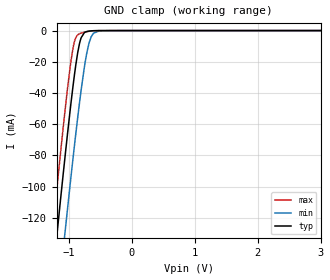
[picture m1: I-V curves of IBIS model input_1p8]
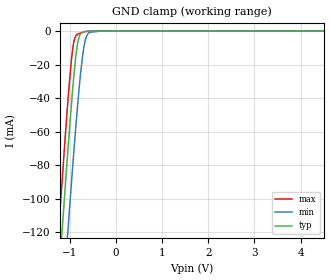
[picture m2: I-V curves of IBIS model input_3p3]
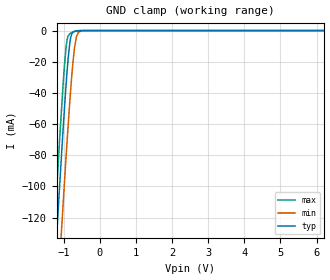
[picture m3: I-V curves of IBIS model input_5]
|Texas Instruments Incorporated
| 12-bit, 8-channel, 1MSPS, SAR ADC with Internal Reference and Internal
| Temperature Sensor
| Marketing part#   Digital Voltage Range   Package-type   #pins
| ADS8028IRTJR   1.65V-5.25V   WQFN   20
| ADS8028IRTJT   1.65V-5.25V   WQFN   20
[IBIS Ver]   4.1
[File name]   ads8028.ibs
[File Rev]   1.0
[Date]   8/3/2015
[Source]
| Texas Instruments Incorporated.
| Analog-eLab Design Center, HPA
| 12500 TI Blvd
| Dallas, TX -75243
[Notes]   Revision History:
| Rev 1.0: 8/3/2015
| - Initial version of the model
| - Model generated from simulations in TISPICE
| - Model matched to SPICE simulation
| - C_comp although listed in numerical order of value are
|   obtained from varying PVT conditions. For PVT conditions for
|   each specific value refer the buffer description under
|   respective [Model]. IBIS model user is responsible for using
|   appropriate C_comp to simulate for Signal Integrity.
[Disclaimer]
| This model is designed as an aid for customers of Texas Instruments.
| TI and its licensors and suppliers make no warranties, either expressed
| or implied, with respect to this  model, including the warranties of
| merchantability or fitness for a particular purpose. The model is
| provided solely on an "as is" basis. The entire risk as to its quality
| and performance is with the customer.
[Copyright]
(C) Copyright 2015 Texas Instruments Incorporated.All rights reserved.
|   ADS8028IRTJ
[Component]   ADS8028IRTJ
[Manufacturer]   TI
[Package]   |20 WQFN - RTJ package
|   typ   min   max
R_pkg   0.06020   0.05752   0.06227
L_pkg   0.91652nH   0.87519nH   0.95139nH
C_pkg   0.12692pF   0.12082pF   0.13078pF
[Pin]  signal_name   model_name   R_pin   L_pin   C_pin
1   AIN3   NC   0.06084   0.93482nH  0.12082pF
2   AIN4   NC   0.05966   0.91410nH  0.12996pF
3   AIN5   NC   0.05964   0.91350nH  0.13005pF
4   AIN6   NC   0.06048   0.92754nH  0.13101pF
5   AIN7   NC   0.06271   0.96574nH  0.12287pF
6   AGND   GND   0.02992   0.59799nH  0.15143pF
7   REF   NC   0.02915   0.57935nH  0.16094pF
8   NC   NC   0.05757   0.87571nH  0.13002pF
9   DGND   GND   0.01969   0.50923nH  0.18030pF
10   AVDD   POWER   0.02967   0.59635nH  0.14994pF
11   _CS   INPUT   0.06227   0.95139nH  0.12238pF
12   TM_BUSY   TRISTATE   0.05995   0.91121nH  0.13014pF
13   DIN   INPUT   0.05966   0.90619nH  0.13006pF
14   DOUT   TRISTATE   0.06040   0.91862nH  0.13078pF
15   SCLK   INPUT   0.06139   0.93650nH  0.12082pF
16   DVDD   POWER   0.06011   0.91724nH  0.11994pF
17   _PD/_RST   INPUT   0.05752   0.87519nH  0.12732pF
18   AIN0   NC   0.05975   0.90986nH  0.12973pF
19   AIN1   NC   0.05767   0.87741nH  0.12809pF
20   AIN2   NC   0.05812   0.88744nH  0.11796pF
|   Model Selectors
[Model Selector] INPUT
input_1p8   1.8V digital Input
input_3p3   3.3V digital Input
input_5   5.0V digital Input
[Model Selector] TRISTATE
tristate_1p8   1.8V digital 3-state
tristate_3p3   3.3V digital 3-state
tristate_5   5.0V digital 3-state
| Models and submodels in the file (6): input_1p8 (Input), input_3p3 (Input), input_5 (Input), tristate_1p8 (3-state), tristate_3p3 (3-state), tristate_5 (3-state)
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|   input_1p8 Model
[Model]   input_1p8
Model_type   Input
Vinl = 0.54
Vinh = 1.26
|   typ   min   max
|   (nom PVT)   (fast PVT)   (slow PVT)
C_comp   4.988e-13   4.299e-13   5.751e-13
[Model spec]
|subparameter
Vinl   0.54   0.495   0.585
Vinh   1.26   1.155   1.365
| Where nom  PVT is Nominal Process, 1.8V, 27C
|   Fast PVT is Strong Process,  1.95V, -40C
|   Slow PVT is Weak Process,   1.65V, 125C
[Voltage Range]   1.8   1.65   1.95
|Junction Temperature
[Temperature Range]   27   125   -40
[Power Clamp Reference]   1.8   1.65   1.95
[GND Clamp Reference]   0   0   0
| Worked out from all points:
|   GND clamp passes 1 mA (typ) near -0.74 V on its own axis
[GND Clamp]
|   Voltage   I(typ)   I(min)   I(max)
-1.8V     -380mA     -425.6mA   -352.6mA
-1.391V   -210.4mA   -258.2mA   -181.1mA
-1.18V    -125.4mA   -174mA     -95.45mA
-1.092V   -91.22mA   -139.8mA   -61.42mA
-1.048V   -74.37mA   -122.7mA   -44.98mA
-937.1mV  -35.3mA    -81.6mA    -11.06mA
-835.2mV  -8.422mA   -46.5mA    -2.027mA
-757.2mV  -1.338mA   -23.42mA   -1.061mA
-684mV    -328.8uA   -8.104mA   -468.9uA
-612mV    -84.34uA   -1.689mA   -138.1uA
-514.7mV  -8.53uA    -159.2uA   -11.73uA
3.6V      0A         0A         0A
[POWER Clamp]
|   Voltage   I(typ)   I(min)   I(max)
-1.8V     0A         0A         0A
0V        0A         0A         0A
3.6V      0A         0A         0A
|   input_3p3 Model
[Model]   input_3p3
Model_type   Input
Vinl = 0.99
Vinh = 2.31
|   typ   min   max
|   (nom PVT)   (fast PVT)   (slow PVT)
C_comp   4.732e-13   4.157e-13   5.388e-13
[Model spec]
|subparameter
Vinl   0.99   0.90   1.08
Vinh   2.31   2.10   2.52
| Where nom  PVT is Nominal Process, 3.3V, 27C
|   Fast PVT is Strong Process,  3.6V, -40C
|   Slow PVT is Weak Process,   3V, 125C
[Voltage Range]   3.3   3   3.6
|Junction Temperature
[Temperature Range]   27   125   -40
[Power Clamp Reference]   3.3   3   3.6
[GND Clamp Reference]   0   0   0
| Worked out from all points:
|   GND clamp passes 1 mA (typ) near -0.74 V on its own axis
[GND Clamp]
|   Voltage   I(typ)   I(min)   I(max)
-3.3V     -1.016A    -1.054A    -993.5mA
-1.611V   -301.2mA   -347.8mA   -273mA
-1.219V   -141mA     -189.5mA   -111.1mA
-1.206V   -135.7mA   -184.3mA   -105.8mA
-1.097V   -93.01mA   -141.6mA   -63.18mA
-1.044V   -73.03mA   -121.3mA   -43.7mA
-915mV    -28.34mA   -73.7mA    -7.024mA
-834mV    -8.217mA   -46.11mA   -2.005mA
-788.7mV  -2.842mA   -32.15mA   -1.387mA
-689.7mV  -363.3uA   -8.982mA   -506.3uA
-579mV    -41.02uA   -756uA     -66.22uA
6.6V      0A         0A         0A
[POWER Clamp]
|   Voltage   I(typ)   I(min)   I(max)
-3.3V     0A         0A         0A
0V        0A         0A         0A
6.6V      0A         0A         0A
|   input_5 Model
[Model]   input_5
Model_type   Input
Vinl = 1.5
Vinh = 3.5
|   typ   min   max
|   (nom PVT)   (fast PVT)   (slow PVT)
C_comp   4.544e-13   4.063e-13   5.101e-13
[Model spec]
|subparameter
Vinl   1.50   1.425   1.575
Vinh   3.50   3.325   3.675
| Where nom  PVT is Nominal Process, 5V, 27C
|   Fast PVT is Strong Process,  5.25V, -40C
|   Slow PVT is Weak Process,   4.75V, 125C
[Voltage Range]   5   4.75   5.25
|Junction Temperature
[Temperature Range]   27   125   -40
[Power Clamp Reference]   5   4.75   5.25
[GND Clamp Reference]   0   0   0
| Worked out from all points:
|   GND clamp passes 1 mA (typ) near -0.74 V on its own axis
[GND Clamp]
|   Voltage   I(typ)   I(min)   I(max)
-5V       -1.743A    -1.775A    -1.725A
-1.267V   -160.2mA   -208.6mA   -130.5mA
-1.195V   -131.5mA   -180mA     -101.5mA
-1.11V    -98.08mA   -146.7mA   -68.21mA
-1.015V   -62.35mA   -110.4mA   -33.59mA
-938.7mV  -35.86mA   -82.21mA   -11.44mA
-900.8mV  -24.09mA   -68.67mA   -5.194mA
-826.3mV  -6.963mA   -43.63mA   -1.876mA
-701.3mV  -445.4uA   -10.94mA   -587uA
-592mV    -54.95uA   -1.039mA   -89.77uA
-460mV    -1.971uA   -40.39uA   -2.112uA
10V       0A         0A         0A
[POWER Clamp]
|   Voltage   I(typ)   I(min)   I(max)
-5V       0A         0A         0A
0V        0A         0A         0A
10V       0A         0A         0A
